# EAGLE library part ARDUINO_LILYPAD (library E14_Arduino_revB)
Device for representing a Lilypad Arduino board with a footprint in an EAGLE design. Created by Dave Young for Element14. More EAGLE documentation at: http://www.element14.com/community/community/knode/cadsoft_eagle
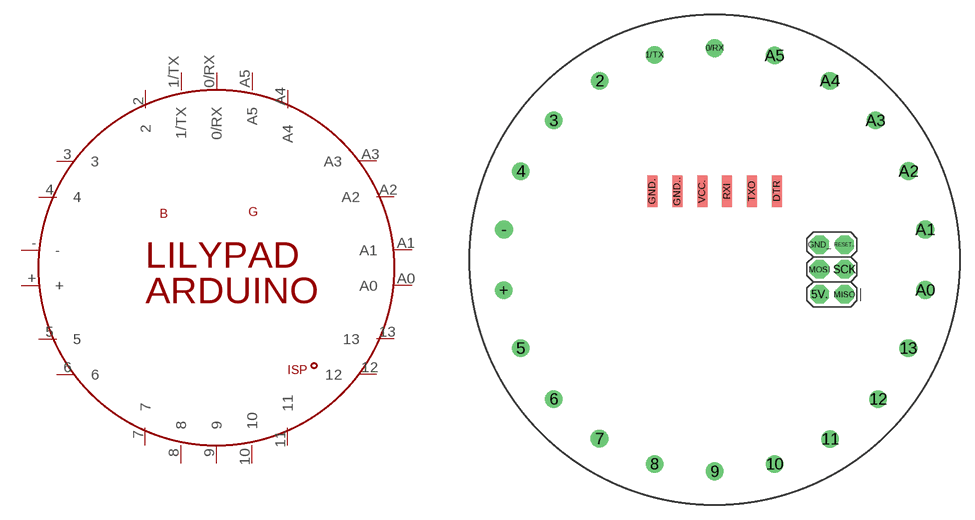
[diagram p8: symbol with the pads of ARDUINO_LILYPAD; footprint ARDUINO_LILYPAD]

Designator prefix PCB

## ARDUINO_LILYPAD  [ARDUINO_LILYPAD]
0/RX  0/RX
1/TX  1/TX
2  2
3  3
4  4
5  5
5V.  VCC
6  6
7  7
8  8
9  9
10  10
11  11
12  12
13  13
+  +
-  -
A0  A0
A1  A1
A2  A2
A3  A3
A4  A4
A5  A5
DTR  DTR
GND.  GND.
GND..  GND..
GND_  GND
MISO  MISO
MOSI  MOSI
RESET..  RST
RXI  RXI
SCK  SCK
TXO  TXO
VCC.  VCC.

## Footprint ARDUINO_LILYPAD (pad centres in mm)
Footprint for representing a Lilypad Arduino board in an EAGLE schematic. Created by Dave Young for Element14. More EAGLE documentation at: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
drill 1.2: 0/RX 0,21.59; 1/TX -6.13,20.89; 2 -11.73,18.26; 3 -16.4,14.21; 4 -19.77,9.03; 5 -19.77,-9.03; 6 -16.4,-14.21; 7 -11.74,-18.26; 8 -6.11,-20.83; 9 0,-21.59; 10 6.11,-20.83; 11 11.76,-18.28; 12 16.654,-14.21; 13 19.74,-9.02; + -21.52,-3.1; - -21.48,3.09; A0 21.48,-3.09; A1 21.48,3.09; A2 19.77,9.04; A3 16.4,14.21; A4 11.74,18.26; A5 6.11,20.83
drill 1.016 pad 1.88 octagon: 5V. 10.693,-3.531; GND_ 10.693,1.549; MISO 13.233,-3.531; MOSI 10.693,-0.991; RESET.. 13.233,1.549; SCK 13.233,-0.991
smd 1.016 x 3.175: DTR 6.35,6.985; GND. -6.35,6.985; GND.. -3.81,6.985; RXI 1.27,6.985; TXO 3.81,6.985; VCC. -1.27,6.985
